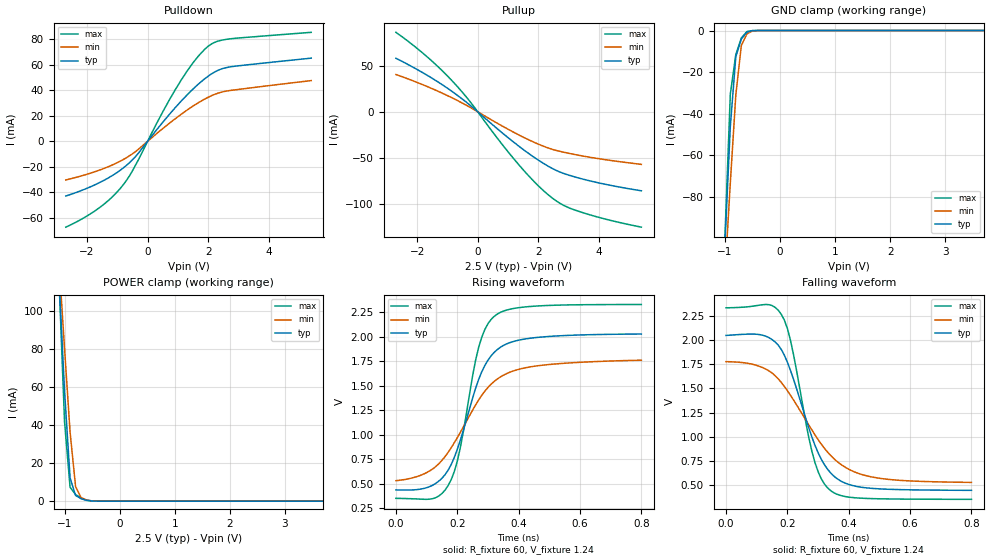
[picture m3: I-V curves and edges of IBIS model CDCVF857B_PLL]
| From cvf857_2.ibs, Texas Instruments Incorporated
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|   Diff. Driver Output  MODEL updated 8/2003
[Model]   CDCVF857B_PLL
Model_type   3-state
Polarity   Non-Inverting
| Signals   FBOUT,FBOUT-,Y0,Y0-, Y1,Y1-, Y2,Y2-, Y3,Y3-, Y4,Y4-,
|   Y5,Y5-, Y6,Y6-, Y7,Y7-, Y8,Y8-, Y9,Y9-
Vmeas = 1.25V   |Vref for timing measurements (crosspoint)
Cref = 14pF   |load capacitance for timing spec (to ground!)
Rref = 60   |60 Ohm to VDD/2 for timing measurements
Vref = 1.25   |Timing specification test load voltage
| variable   typ   min   max
C_comp   2.4pF   2.0pF   2.7pF
[Temperature Range]   40.0   105   0
[Voltage range]   2.5V   2.3V   2.7V
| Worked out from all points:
|   slope of the pulldown table from 0 to 0.375 V, typ, clamps not added: 33.3 ohm
|   slope of the pullup table from 0 to 0.375 V, typ, clamps not added: 34.6 ohm
|   GND clamp passes 1 mA (typ) near -0.61 V on its own axis
|   POWER clamp passes 1 mA (typ) near -0.67 V on its own axis
|   rising waveform, R_fixture 60, V_fixture 1.24: 20-80 % time 102ps typ, 150ps min, 72.5ps max; typ from 0.438 V to 2.03 V
|   falling waveform, R_fixture 60, V_fixture 1.24: 20-80 % time 106ps typ, 162ps min, 74.5ps max; typ from 2.05 V to 0.447 V
[Pullup]
|   40C:2.5V:nominal 105C:2.3V:weak   0C:2.7V:strong
|   Voltage   I(typ)   I(min)   I(max)
-2.7V     58.06mA    40.49mA    86.29mA
-1.7V     40.25mA    27.85mA    60.54mA
-900mV    23.3mA     15.98mA    35.5mA
-300mV    8.384mA    5.704mA    12.94mA
700mV     -19.95mA   -13.47mA   -30.93mA
1.3V      -35.9mA    -24.18mA   -55.38mA
1.9V      -50.31mA   -33.72mA   -77.12mA
2.4V      -60.47mA   -40.15mA   -92.13mA
2.8V      -66.59mA   -43.63mA   -101mA
3.3V      -71.64mA   -47.04mA   -107.8mA
4.2V      -78.68mA   -51.97mA   -116.4mA
5.4V      -85.8mA    -57.13mA   -125.3mA
[Pulldown]
|   40C:2.5V:nominal   105C:2.3V:weak   0C:2.7V:strong
|   Voltage   I(typ)   I(min)   I(max)
-2.7V     -42.96mA   -30.37mA   -67.38mA
-1.6V     -32.59mA   -22.72mA   -52.28mA
-1.2V     -27.42mA   -18.96mA   -44.42mA
-800mV    -20.89mA   -14.29mA   -34.01mA
-400mV    -12.02mA   -8.101mA   -18.78mA
500mV     14.9mA     9.979mA    23.08mA
1.1V      31.31mA    21.04mA    47.7mA
1.5V      41.03mA    27.64mA    61.59mA
2V        51.1mA     34.55mA    74.57mA
2.3V      55.4mA     37.56mA    78.41mA
2.7V      58.27mA    39.76mA    80.29mA
5.4V      65.21mA    47.59mA    85.47mA
[GND Clamp]
|   40C:2.5V:nominal  105C:2.3V:weak   0C:2.7V:strong
|  Voltage   I(typ)   I(min)   I(max)
-2.7V     -1.103A    -887.8mA   -1.395A
-1.1V     -162.1mA   -163.9mA   -171.8mA
-900mV    -46.23mA   -73.5mA    -30.7mA
-800mV    -12.6mA    -30.96mA   -11.52mA
-700mV    -4.108mA   -7.28mA    -3.616mA
-600mV    -807.7uA   -1.647mA   -496.6uA
-500mV    -81.09uA   -268.7uA   -30.08uA
-300mV    -219.6nA   -2.842uA   -15.58nA
5.4V      252.8pA    5.148nA    125.2pA
[POWER Clamp]
|   40C:2.5V:nominal   105C:2.3V:weak   0C:2.7V:strong
|  Voltage   I(typ)   I(min)   I(max)
-2.7V     1.057A     849.3mA    1.339A
-1.1V     116.1mA    125.3mA    115.7mA
-1V       57.76mA    80.13mA    41.69mA
-900mV    12.21mA    36.35mA    7.299mA
-800mV    2.976mA    7.713mA    3.48mA
-700mV    1.27mA     1.885mA    1.613mA
-600mV    407.8uA    568.5uA    461.4uA
-400mV    5.905uA    16.46uA    4.279uA
5.4V      0A         0A         0A
[ramp]
| variable   typ   min   max
dV/dt_r   0.9566/1.0240E-10   0.7468/1.5201E-10   1.1331/6.9055E-11
dV/dt_f   0.9566/1.0535E-10   0.7468/1.6224E-10   1.1331/6.9424E-11
[Rising Waveform]
R_fixture = 60
V_fixture = 1.24
V_fixture_min = 1.14
V_fixture_max = 1.39
| The start delay in the PLL-Type Model does not represent the phase between
| CLOCK and Yx. It has been set to its minimum value to plot the transitions.
| However, the shift in TPD between TYP/WEAK/STRONG has been minimized as it
| perfroms on a locked PLL.
|   40C:2.5V:nominal  105C:2.3V:weak   0C:2.7V:strong
|   Time   V(typ)   V(min)   V(max)
0s        437.6mV    531.9mV    351.5mV
110ps     471.3mV    631.9mV    343.2mV
170ps     638.1mV    820.9mV    481mV
190ps     767.1mV    918.3mV    621.6mV
210ps     945.3mV    1.026V     870.4mV
270ps     1.569V     1.358V     1.898V
290ps     1.71V      1.447V     2.077V
320ps     1.841V     1.545V     2.209V
440ps     1.988V     1.696V     2.312V
800ps     2.03V      1.763V     2.332V
[Falling Waveform]
R_fixture = 60
V_fixture = 1.24
V_fixture_min = 1.14
V_fixture_max = 1.39
|   40C:2.5V:nominal   105C:2.3V:weak  0C:2.7V:strong
|   Time   V(typ)   V(min)   V(max)
0s        2.048V     1.777V     2.334V
120ps     2.05V      1.715V     2.366V
180ps     1.904V     1.563V     2.267V
210ps     1.687V     1.43V      1.998V
270ps     1.089V     1.121V     988.3mV
290ps     911.2mV    1.02V      732.8mV
340ps     630.1mV    810.7mV    446.3mV
390ps     519.4mV    682.5mV    382.1mV
480ps     466.4mV    582.3mV    361.2mV
800ps     447mV      529.1mV    354.1mV
